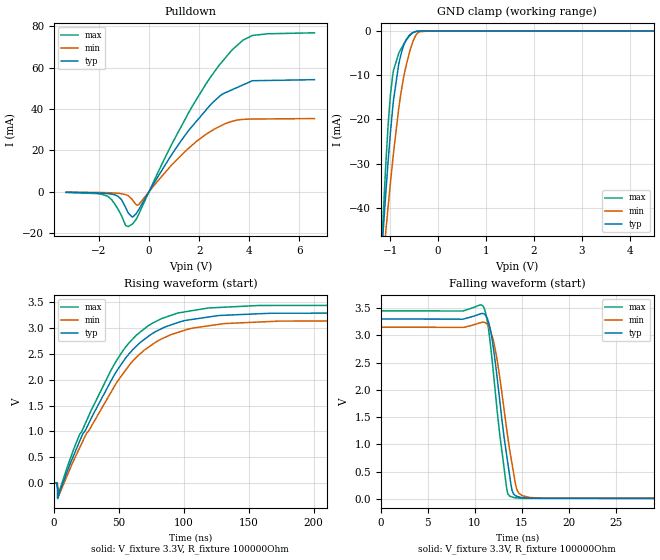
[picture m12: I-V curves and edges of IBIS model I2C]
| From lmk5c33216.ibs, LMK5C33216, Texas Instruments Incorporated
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|   I2C Model
[Model]   I2C
Model_type   I/O_open_drain
Polarity   Non-Inverting
Enable   Active-Low
Vinl = 0.6
Vinh = 1.2
Vmeas = 1.65
Vref = 3.3
Cref = 2pF
Rref = 100000
|   typ   min   max
C_comp   2.1556E-13  2.1055E-13   2.4065E-13
| Where nom  PVT is Nominal Process, 3.3V,   27C
|   Fast PVT is Strong Process,  3.45V, -40C
|   Slow PVT is Weak Process,   3.15V, 125C
[Model spec]
|subparameter
Vinl   0.6   0.57   0.63
Vinh   1.2   1.15   1.25
[Voltage Range]   3.3   3.15   3.45
|Junction Temperature
[Temperature Range]   27   125   -40
[Pullup Reference]   3.3   3.15   3.45
[Pulldown Reference]   -0   0   -0
[Power Clamp Reference]   3.3   3.15   3.45
[GND Clamp Reference]   0   0   0
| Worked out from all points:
|   slope of the pulldown table from 0 to 0.495 V, typ, clamps not added: 49.5 ohm
|   GND clamp passes 1 mA (typ) near -0.61 V on its own axis
|   falling waveform, V_fixture 3.3V, R_fixture 100000Ohm: 20-80 % time 1.43ns typ, 1.57ns min, 1.31ns max; typ from 3.3 V to 0.002 V
|   rising waveform, V_fixture 3.3V, R_fixture 100000Ohm: 20-80 % time 45.7ns typ, 48.3ns min, 43.8ns max; typ from 0.002 V to 3.3 V
[Pulldown]
|   Voltage   I(typ)   I(min)   I(max)
-3.3V     -255.7uA   -171.8uA   -331.7uA
-1.649V   -889.5uA   -451.9uA   -2.109mA
-1.244V   -2.112mA   -722.7uA   -8.228mA
-930.6mV  -7.583mA   -1.361mA   -16.34mA
-666.8mV  -12.22mA   -3.757mA   -15.64mA
-393.5mV  -8.323mA   -6.002mA   -10.45mA
714mV     14.28mA    10.3mA     18.27mA
1.62V     30.24mA    21.45mA    39.08mA
2.685V    44.75mA    30.79mA    59.28mA
3.303V    49.26mA    34.02mA    68.43mA
4.125V    53.7mA     35.17mA    75.56mA
6.6V      54.19mA    35.39mA    76.85mA
[GND Clamp]
|   Voltage   I(typ)   I(min)   I(max)
-3.3V     -455.8mA   -344.6mA   -657.3mA
-1.161V   -47.31mA   -53.45mA   -44.68mA
-1.095V   -36.77mA   -45.47mA   -30.31mA
-996.7mV  -22.95mA   -34.32mA   -14.44mA
-945.4mV  -16.96mA   -28.87mA   -9.725mA
-824.9mV  -7.572mA   -17.64mA   -5.071mA
-774.7mV  -5.214mA   -13.86mA   -4.013mA
-669.3mV  -1.98mA    -7.818mA   -2.116mA
-517.7mV  -289.6uA   -2.119mA   -331uA
-426.8mV  -45.38uA   -439.6uA   -41.41uA
-194.7mV  -4.022uA   -4.73uA    -4.478uA
6.6V      0A         0A         0A
[POWER Clamp]
|   Voltage   I(typ)   I(min)   I(max)
-3.3V     0A         0A         0A
0V        0A         0A         0A
6.6V      0A         0A         0A
[Ramp]
R_load = 100000
|   typ   min   max
dV/dt_r   1.97895/4.58324e-08   1.88832/4.84345e-08   2.06912/4.37125e-08
dV/dt_f   1.97895/1.42783e-09   1.88832/1.56573e-09   2.06912/1.31234e-09
[Falling Waveform]
V_fixture = 3.3V
V_fixture_min = 3.15V
V_fixture_max = 3.45V
R_fixture = 100000Ohm
C_fixture = 0F
|   Time   V(typ)   V(min)   V(max)
0s        3.3V       3.149V     3.45V
10.92ns   3.398V     3.241V     3.524V
11.39ns   3.281V     3.19V      3.198V
12.08ns   2.638V     2.826V     2.138V
13.43ns   748.4mV    1.223V     149.4mV
13.94ns   170.2mV    655.9mV    34.98mV
14.26ns   66.44mV    337.8mV    18.8mV
15.01ns   21.34mV    60.21mV    8.075mV
17.07ns   8.783mV    11.27mV    8.047mV
100ns     1.732mV    2.234mV    1.448mV
[Rising Waveform]
V_fixture = 3.3V
V_fixture_min = 3.15V
V_fixture_max = 3.45V
R_fixture = 100000Ohm
C_fixture = 0F
|   Time   V(typ)   V(min)   V(max)
0s        1.732mV    2.234mV    1.448mV
2.367ns   2.365mV    2.649mV    2.199mV
2.918ns   -95.67mV   -38.33mV   -302.2mV
3.776ns   -238.2mV   -245.4mV   -194.6mV
19.56ns   790.7mV    665.7mV    923.4mV
52.61ns   2.325V     2.095V     2.542V
72.07ns   2.827V     2.616V     3.036V
94.39ns   3.098V     2.908V     3.285V
173.4ns   3.289V     3.137V     3.44V
500ns     3.3V       3.149V     3.45V
